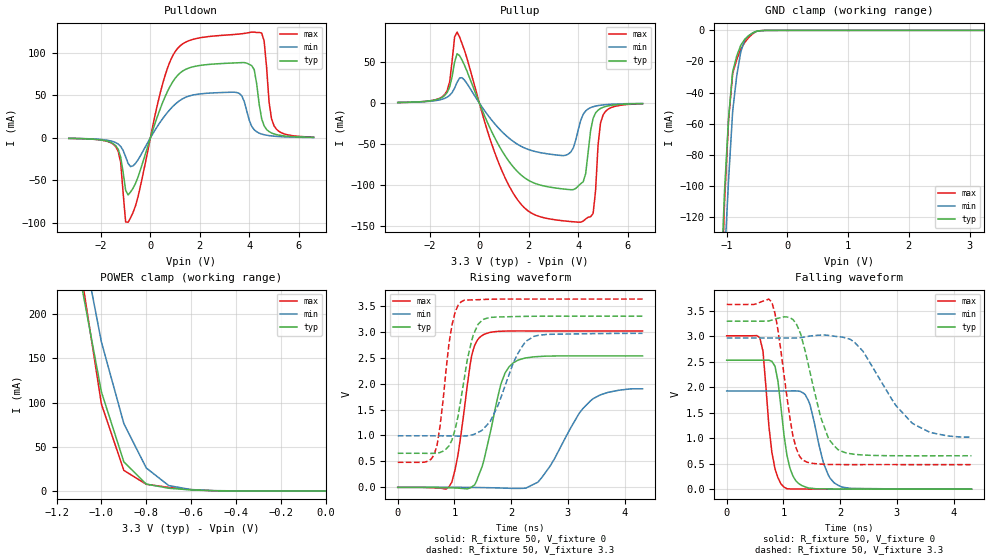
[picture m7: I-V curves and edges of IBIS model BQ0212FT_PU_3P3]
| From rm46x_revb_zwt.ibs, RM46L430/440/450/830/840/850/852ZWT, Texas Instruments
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|   Model Cell BQ0212FT_PU_3P3
|BQ0212FT_PU_3P3
[Model]   BQ0212FT_PU_3P3
Model_type   I/O
Polarity   Non-Inverting
Enable   Active-Low
Vinl =  1.15
Vinh =  1.55
Cref =  15.0001pF
Rref =  101.0000M
Vref =  0V
Vmeas =  1.65
C_comp   1.2p   1.2p   1.2p
[Model Spec]
Vinl   1.15   1.02   1.28
Vinh   1.55   1.45   1.65
[Temperature Range]   25   155   -40
[Voltage Range]   3.3   2.97   3.63
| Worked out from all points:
|   slope of the pulldown table from 0 to 0.495 V, typ, clamps not added: 11.9 ohm
|   slope of the pullup table from 0 to 0.495 V, typ, clamps not added: 14.3 ohm
|   GND clamp passes 1 mA (typ) near -0.53 V on its own axis
|   POWER clamp passes 1 mA (typ) near -0.59 V on its own axis
|   rising waveform, R_fixture 50, V_fixture 0: 20-80 % time 315ps typ, 599ps min, 226ps max; typ from 0 V to 2.53 V
|   rising waveform, R_fixture 50, V_fixture 3.3: 20-80 % time 266ps typ, 432ps min, 201ps max; typ from 0.657 V to 3.3 V
|   falling waveform, R_fixture 50, V_fixture 0: 20-80 % time 182ps typ, 257ps min, 155ps max; typ from 2.53 V to 0 V
|   falling waveform, R_fixture 50, V_fixture 3.3: 20-80 % time 362ps typ, 700ps min, 238ps max; typ from 3.3 V to 0.657 V
[POWER_clamp]
|   voltage   I(typ)   I(min)   I(max)
-3.3V     4.054A     4.63A      4.887A
-1.1V     248.3mA    301mA      262.7mA
-1.067V   202.9mA    256.9mA    207.9mA
-1.033V   157.5mA    212.7mA    153.1mA
-1V       112.1mA    168.6mA    98.31mA
-900mV    32.89mA    76.23mA    23.24mA
-800mV    7.72mA     25.95mA    7.497mA
-700mV    3.046mA    6.046mA    4.01mA
-600mV    1.099mA    1.535mA    1.442mA
-500mV    196.6uA    374.7uA    217.1uA
0V        442.6pA    6.158nA    416.6pA
[Pulldown]
|   voltage   I(typ)   I(min)   I(max)
-3.3V     -593uA     -522.6uA   -580.3uA
-1.4V     -9.188mA   -5.565mA   -10.35mA
-1.2V     -22.55mA   -10.08mA   -29.13mA
-1V       -61.66mA   -22.23mA   -99.07mA
-900mV    -67.21mA   -30.1mA    -99.29mA
1V        70.16mA    39.61mA    101.5mA
3.5V      88.44mA    53.41mA    122.1mA
4.2V      80.27mA    9.542mA    124.6mA
4.6V      14.18mA    3.749mA    114.2mA
4.8V      7.418mA    2.695mA    42.04mA
5V        4.687mA    2.03mA     14.29mA
6.6V      680.4uA    493.7uA    947.4uA
[Pullup]
|   voltage   I(typ)   I(min)   I(max)
-3.3V     671.9uA    618.2uA    613.1uA
-1.4V     9.171mA    5.687mA    10.35mA
-900mV    59.98mA    25.21mA    86.36mA
600mV     -40.93mA   -24.46mA   -58.45mA
1.4V      -78.76mA   -47.34mA   -111.2mA
3.5V      -105mA     -63.56mA   -143.7mA
4.1V      -98.17mA   -21.1mA    -145.1mA
4.3V      -85.91mA   -9.61mA    -141.1mA
4.6V      -18.69mA   -4.516mA   -134.6mA
4.8V      -8.691mA   -3.128mA   -51.49mA
5V        -5.242mA   -2.297mA   -14.81mA
6.6V      -711.8uA   -541.3uA   -921.2uA
[GND_clamp]
|   voltage   I(typ)   I(min)   I(max)
-3.3V     -3.25A     -2.875A    -4.945A
-1.1V     -166.9mA   -205.1mA   -187mA
-1.033V   -102.8mA   -146.7mA   -110.1mA
-966.7mV  -55.96mA   -95.69mA   -57.02mA
-900mV    -26.55mA   -52.03mA   -27.8mA
-833.3mV  -16.5mA    -29.28mA   -18.78mA
-766.7mV  -9.55mA    -13.91mA   -12.09mA
-700mV    -5.706mA   -5.929mA   -7.734mA
-566.7mV  -1.585mA   -1.639mA   -2.086mA
-500mV    -421.6uA   -604.2uA   -492.4uA
-366.7mV  -38.21uA   -69.49uA   -50.21uA
3.233V    -1.13uA    7.006uA    -9.303uA
[Ramp]
| variable   typ   min   max
dV/dt_f   1.638098/0.373132n   1.223096/0.7334904n   1.953602/0.2453702n
dV/dt_r   1.539983/0.3181168n   1.172113/0.6247548n   1.831174/0.2271902n
R_load = 50
[Rising Waveform]
R_fixture = 50
V_fixture = 0
V_fixture_min = 0
V_fixture_max = 0
|   time   V(typ)   V(min)   V(max)
0s        163.1uV    141.6uV    188.3uV
956ps     -9.711mV   343uV      106.2mV
1.064ns   -15.13mV   272.4uV    637.2mV
1.304ns   7.871mV    -1.808mV   2.539V
1.468ns   346.8mV    -4.119mV   2.913V
1.82ns    1.995V     -12.58mV   3.009V
2.036ns   2.4V       -21.01mV   3.015V
2.472ns   2.521V     100.4mV    3.015V
3.444ns   2.534V     1.708V     3.014V
4.316ns   2.534V     1.9V       3.014V
[Rising Waveform]
R_fixture = 50
V_fixture = 3.3
V_fixture_min = 2.97
V_fixture_max = 3.63
|   time   V(typ)   V(min)   V(max)
0s        656.9mV    993.5mV    482.7mV
640ps     655.8mV    993.5mV    623.9mV
744ps     671.2mV    993.3mV    1.163V
956ps     911.8mV    990.5mV    3.127V
1.116ns   1.713V     988.2mV    3.575V
1.332ns   2.936V     1.017V     3.614V
1.52ns    3.243V     1.139V     3.622V
2.108ns   3.294V     2.561V     3.63V
2.4ns     3.298V     2.91V      3.63V
4.316ns   3.3V       2.969V     3.63V
[Falling Waveform]
R_fixture = 50
V_fixture = 0
V_fixture_min = 0
V_fixture_max = 0
|   time   V(typ)   V(min)   V(max)
0s        2.534V     1.93V      3.014V
584ps     2.534V     1.93V      2.975V
640ps     2.534V     1.93V      2.711V
852ps     2.415V     1.93V      398.2mV
1.012ns   1.047V     1.93V      38.5mV
1.224ns   157.9mV    1.931V     4.378mV
1.44ns    24.38mV    1.74V      2.179mV
1.712ns   5.381mV    493.9mV    749.4uV
1.964ns   3.006mV    76.54mV    496.8uV
4.316ns   262.2uV    941.6uV    194.3uV
[Falling Waveform]
R_fixture = 50
V_fixture = 3.3
V_fixture_min = 2.97
V_fixture_max = 3.63
|   time   V(typ)   V(min)   V(max)
0s        3.3V       2.97V      3.63V
796ps     3.322V     2.97V      3.674V
904ps     3.358V     2.97V      3.128V
1.168ns   3.334V     2.97V      1.046V
1.332ns   2.932V     2.983V     578.1mV
1.656ns   1.418V     3.027V     492.9mV
1.964ns   775.6mV    2.996V     483.3mV
2.4ns     671.8mV    2.714V     482.8mV
3.268ns   655.9mV    1.299V     482.8mV
4.316ns   656.7mV    1.024V     482.7mV
